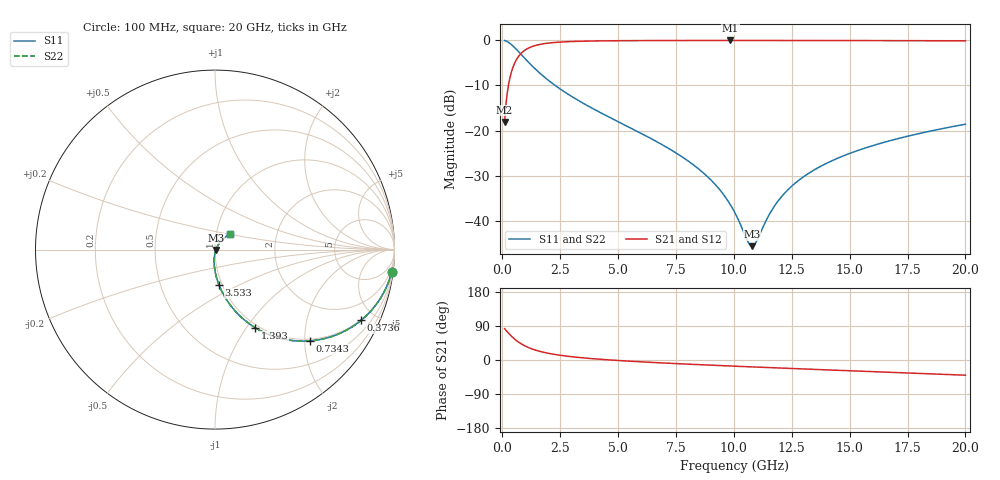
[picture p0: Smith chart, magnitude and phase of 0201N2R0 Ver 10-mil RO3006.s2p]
# GHz S MA R 50
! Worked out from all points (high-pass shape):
!   1601 points, 100 MHz to 20 GHz, reference 50 ohm
!   highest |S21| = -0.05 dB at 9.851 GHz (marker M1); lowest = -18.1 dB at 100 MHz (marker M2)
!   |S21| within 3 dB of the highest: 787 MHz to end of sweep
!   lowest |S11| = -45.6 dB at 10.78 GHz (marker M3), VSWR 1.01, Z = 50.5 - j0.178 ohm
!   |S11| at or under -10 dB: 2.28 GHz to end of sweep
!   |S22| runs from -45.6 to -0.1 dB; largest |S21 - S12| = 0
!   S11 on the Smith chart (normalised r, x): 100 MHz: 1, -16; 373.6 MHz: 0.96, -4.16; 734.3 MHz: 0.96, -2.11; 1.393 GHz: 0.96, -1.10; 3.533 GHz: 0.97, -0.40; 20 GHz: 1.16, +0.20
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0.1  0.9922 -7.3  0.1247 82.6  0.1247 82.6  0.9922 -7.3
0.2616875  0.9497 -18.7  0.3125 71.3  0.3125 71.3  0.9497 -18.7
0.373625  0.9046 -25.8  0.4253 64.1  0.4253 64.1  0.9046 -25.8
0.7343125  0.7325 -44.0  0.679 45.8  0.679 45.8  0.7325 -44.0
1.04525  0.6012 -54.6  0.7969 35.2  0.7969 35.2  0.6012 -54.6
1.3935  0.4889 -62.8  0.8698 26.9  0.8698 26.9  0.4889 -62.8
2.177062  0.3307 -73.9  0.9407 15.6  0.9407 15.6  0.3307 -73.9
3.420812  0.2055 -83.0  0.9751 6.0  0.9751 6.0  0.2055 -83.0
3.53275  0.1979 -83.6  0.9766 5.4  0.9766 5.4  0.1979 -83.6
6.741625  0.07351 -93.8  0.9927 -7.2  0.9927 -7.2  0.07351 -93.8
8.657  0.03438 -94.7  0.9944 -12.7  0.9944 -12.7  0.03438 -94.7
9.851  0.01505 -86.2  0.9946 -15.9  0.9946 -15.9  0.01505 -86.2
10.05  0.0122 -81.7  0.9946 -16.4  0.9946 -16.4  0.0122 -81.7
10.59725  0.005934 -46.6  0.9945 -17.8  0.9945 -17.8  0.005934 -46.6
10.78381  0.005235 -19.7  0.9945 -18.2  0.9945 -18.2  0.005235 -19.7
10.95794  0.005779 5.6  0.9945 -18.7  0.9945 -18.7  0.005779 5.6
11.51763  0.01159 42.3  0.9943 -20.0  0.9943 -20.0  0.01159 42.3
11.99025  0.01761 50.7  0.9941 -21.2  0.9941 -21.2  0.01761 50.7
13.37081  0.03535 56.2  0.9933 -24.5  0.9933 -24.5  0.03535 56.2
14.80113  0.05326 55.6  0.9923 -27.9  0.9923 -27.9  0.05326 55.6
16.69162  0.0765 52.9  0.9904 -32.4  0.9904 -32.4  0.0765 52.9
20  0.1175 46.5  0.9857 -40.1  0.9857 -40.1  0.1175 46.5
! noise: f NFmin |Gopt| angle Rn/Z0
0.1  0.000962  0.9563  0.6412  0.004955
2.301  0.005358  0.8259  4.267  0.006462
4.515  0.008286  0.7843  7.93  0.007855
6.729  0.01081  0.7577  11.59  0.008937
8.943  0.01311  0.7382  15.23  0.009854
11.14  0.01527  0.7232  18.82  0.01066
13.36  0.01735  0.7111  22.4  0.0114
15.57  0.01937  0.7014  25.94  0.01208
17.79  0.02134  0.6935  29.43  0.01273
20  0.02329  0.6871  32.88  0.01334
